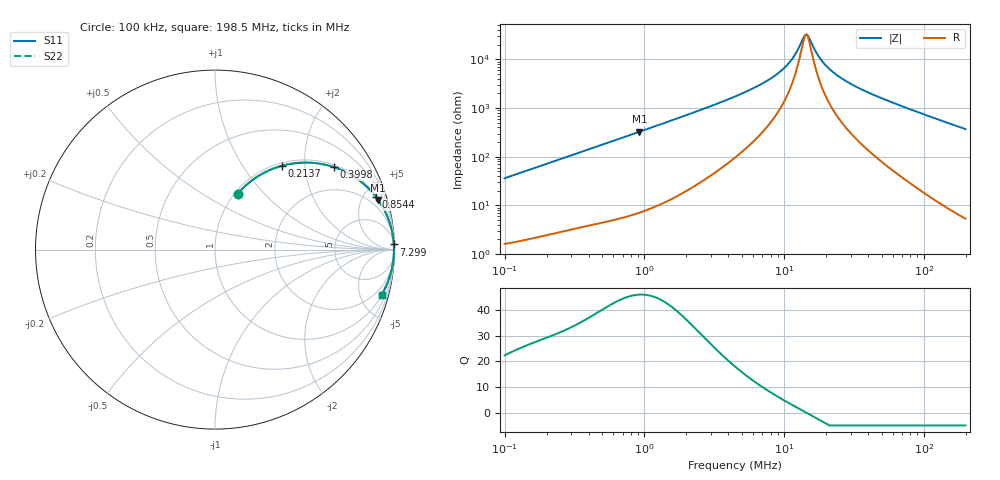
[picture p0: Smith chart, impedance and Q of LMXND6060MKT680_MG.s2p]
! LMXND6060MKT680_MG  S-PARAMETER MODEL  ( General Type )
! Model Generated by TAIYO YUDEN Corporation (http://www.ty-top.com)
! Version 1.0
! TAIYO YUDEN Control No. 191025NI43SB-FBB
! Copyright(c) 2019 TAIYO YUDEN CO.,LTD. All Rights Reserved.
! Product Description (link to TY-COMPAS)
! https://ds.yuden.co.jp/TYCOMPAS/or/detail?pn=LMXND6060MKT680MMG&u=M
! Products Name : Inductors
! Characteristics :
!  Inductance : 68 uH , SRF(min) : 3.0 MHz , DC Resistance(max) : 1.392 Ohm
!  Rated Current : Saturation :440 mA , Temp Rise : 410 mA
!  Case Size : 6.0 x 6.0 / 0.236 x 0.236 [mm/inch] , Thickness : 1.2 / 0.047 [mm/inch]
!  (Conditions: Temperature = 25 degC , DC Bias Current/Voltage = 0A / 0V)
! External Node Assignments :
!  1  o---GGG---o  2
! GND o---------o GND
! Frequency Range : 0.1MHz  -  198.534594MHz  [ 402 STEP ]
# MHz S RI R 50
! Freq[MHz].  S11 Real  S11 Imag  S21 Real  S21 Imag  S12 Real  S12 Imag  S22 Real  S22 Imag
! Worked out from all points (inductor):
!   401 points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, 100 kHz to 198.5 MHz, reference 50 ohm
!   read as one part in series: L = 57.3 uH near 103.9 kHz
!   highest Q = 46 at 921.8 kHz (marker M1), where L = 56.2 uH
!   self-resonance near 14.19 MHz
!   S11 on the Smith chart (normalised r, x): 100 kHz: 1.03, +0.72; 213.7 kHz: 1.05, +1.53; 399.8 kHz: 1.08, +2.84; 854.4 kHz: 1.13, +6.04; 7.299 MHz: 8, +68; 198.5 MHz: 1.11, -7.39
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0.1  0.1262 0.3104  0.8738 -0.3104  0.8738 -0.3104  0.1262 0.3104
0.143432  0.2192 0.3951  0.7808 -0.3951  0.7808 -0.3951  0.2192 0.3951
0.21369  0.3733 0.4672  0.6267 -0.4672  0.6267 -0.4672  0.3733 0.4672
0.356769  0.6132 0.4731  0.3868 -0.4731  0.3868 -0.4731  0.6132 0.4731
0.399811  0.6637 0.4591  0.3363 -0.4591  0.3363 -0.4591  0.6637 0.4591
0.854356  0.896 0.2946  0.104 -0.2946  0.104 -0.2946  0.896 0.2946
0.921758  0.9089 0.2771  0.0911 -0.2771  0.0911 -0.2771  0.9089 0.2771
1.272844  0.9489 0.2093  0.0511 -0.2093  0.0511 -0.2093  0.9489 0.2093
4.541117  0.9937 0.0559  0.00634 -0.0559  0.00634 -0.0559  0.9937 0.0559
7.299237  0.9961 0.0288  0.00393 -0.0288  0.00393 -0.0288  0.9961 0.0288
8.994312  0.9965 0.0192  0.00345 -0.0192  0.00345 -0.0192  0.9965 0.0192
10.67012  0.9968 0.012  0.00321 -0.012  0.00321 -0.012  0.9968 0.012
11.9574  0.9969 0.00739  0.00312 -0.00739  0.00312 -0.00739  0.9969 0.00739
14.18529  0.9969 0.000638  0.00306 -0.000638  0.00306 -0.000638  0.9969 0.000638
15.01661  0.9969 -0.0016  0.00306 0.0016  0.00306 0.0016  0.9969 -0.0016
15.89665  0.9969 -0.00384  0.00307 0.00384  0.00307 0.00384  0.9969 -0.00384
17.15079  0.9969 -0.00685  0.0031 0.00685  0.0031 0.00685  0.9969 -0.00685
18.85849  0.9968 -0.0107  0.00317 0.0107  0.00317 0.0107  0.9968 -0.0107
23.68329  0.9965 -0.0203  0.00347 0.0203  0.00347 0.0203  0.9965 -0.0203
33.33072  0.9956 -0.0368  0.00443 0.0368  0.00443 0.0368  0.9956 -0.0368
56.71438  0.9917 -0.0718  0.00831 0.0718  0.00831 0.0718  0.9917 -0.0718
198.5346  0.9287 -0.2502  0.0713 0.2502  0.0713 0.2502  0.9287 -0.2502
